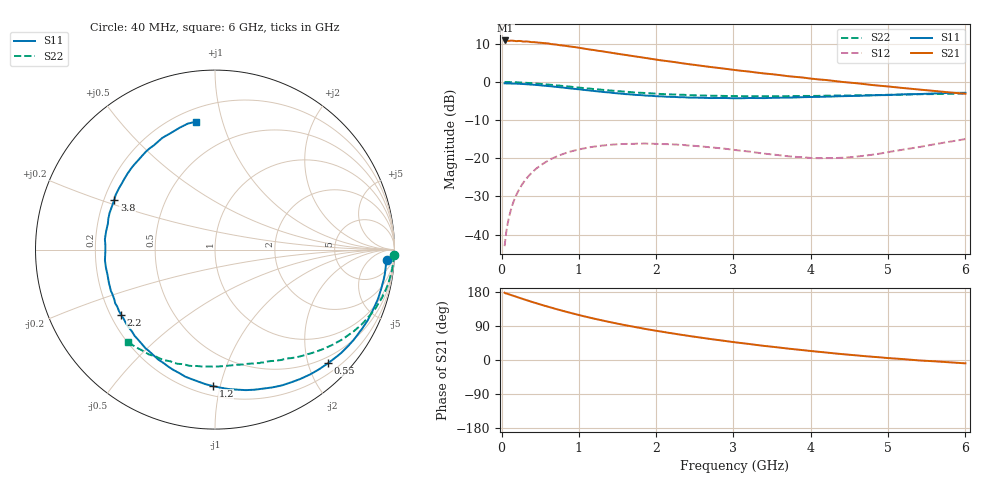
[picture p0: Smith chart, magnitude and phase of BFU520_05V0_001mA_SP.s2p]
! Filename:  P:\Prog\Test\Noise\ATS_data\Testdata_Net\03 Spar\BFU520_APG2013_37_A05_05p0V_001mA_SP_CM01_D.s2p
! Date/Time: Fri 26/Apr/2013 13:00:07
! BFU520_APG2013_37_A05_05p0V_1to20mA_SP_CM01_Bias1_R.s2p
! MDIF S-parameter v. bias file
! BFU520_APG2013_37_A05_05p0V_1to20mA_SP_CM01
! Date/time Tue Apr 23 15:26:19 2013
! bias mode 1
! bias variable = I_out
! VAR bias_var= 1
! VAR V_out= 5.0000
! VAR I_out= 1.0000
! VAR V_in= 0.7910
! VAR I_in= 0.0110
! Device data file deembeded for feedlines and parallel
! Original file: \03 Spar\BFU520_APG2013_37_A05_05p0V_001mA_SP_CM01_R.s2p
! Feed-files: PR047V01_250413_Feed1.s2p, PR047V01_250413_Feed2.s2p
! Parallel-file: PR047V01_250413_Par.s2p
# MHz S MA R 50
!  Freq-MHz  S11-mag  S11-arg  S21-mag  S21-arg  S12-mag  S12-arg  S22-mag  S22-arg
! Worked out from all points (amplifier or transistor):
!   98 points, 40 MHz to 6 GHz, reference 50 ohm
!   highest |S21| = 10.9 dB at 50 MHz (marker M1)
!   |S21| within 3 dB of that: start of sweep to 1.349 GHz
!   unconditionally stable (mu >= 1): 3.506 GHz to 5.262 GHz
!   at 300 MHz: K = 0.08, MSG = 18.3 dB, |S12| = -25.9 dB
!   at 1.6 GHz: K = 0.39, MSG = 11.7 dB, |S12| = -16.3 dB
!   at 6 GHz: K = 0.82, MSG = 5.9 dB, |S12| = -15.0 dB
!   S11 on the Smith chart (normalised r, x): 40 MHz: 16, -22; 550 MHz: 0.38, -2.36; 1.2 GHz: 0.26, -0.95; 2.2 GHz: 0.24, -0.30; 3.8 GHz: 0.24, +0.22; 6 GHz: 0.28, +0.82
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40  0.9585 -3.4  3.493 177.5  0.007033 87.2  0.9973 -1.7
50  0.9574 -4.2  3.499 176.0  0.00869 87.1  0.9989 -2.1
100  0.9559 -8.3  3.453 173.1  0.01739 84.3  0.9953 -4.4
120  0.9545 -10.1  3.484 171.7  0.0208 83.3  0.9937 -5.3
200  0.9492 -16.6  3.428 166.2  0.03442 78.7  0.9879 -9.0
240  0.9433 -20.1  3.446 163.5  0.04099 76.6  0.9844 -10.7
340  0.9308 -28.2  3.385 156.8  0.05681 71.3  0.9707 -15.1
550  0.8931 -45.1  3.228 143.6  0.08633 60.6  0.9342 -23.6
700  0.8635 -56.5  3.098 134.8  0.1039 53.7  0.9049 -29.1
800  0.8435 -63.8  2.999 129.3  0.114 49.5  0.8835 -32.5
1050  0.7897 -81.1  2.757 116.2  0.1336 39.7  0.8338 -40.3
1200  0.7603 -90.9  2.615 109.0  0.142 34.5  0.8062 -44.4
1600  0.6934 -114.7  2.265 91.8  0.1539 22.7  0.7447 -54.0
1850  0.6648 -128.0  2.072 82.4  0.1559 16.9  0.7172 -59.1
2050  0.6474 -137.8  1.928 75.5  0.1535 12.9  0.6962 -63.0
2200  0.6376 -145.0  1.844 70.6  0.1522 10.3  0.6867 -65.7
2600  0.6193 -162.7  1.621 58.4  0.1421 4.8  0.6642 -73.1
3100  0.6116 177.6  1.402 44.8  0.1254 2.2  0.6516 -81.7
3800  0.6261 153.6  1.166 28.1  0.1043 8.5  0.6531 -93.9
4100  0.637 144.3  1.08 21.7  0.1001 15.0  0.6566 -99.2
5200  0.6882 115.3  0.8317 2.3  0.1299 37.5  0.681 -118.8
6000  0.7209 98.4  0.7007 -8.8  0.1782 39.9  0.7058 -133.4
